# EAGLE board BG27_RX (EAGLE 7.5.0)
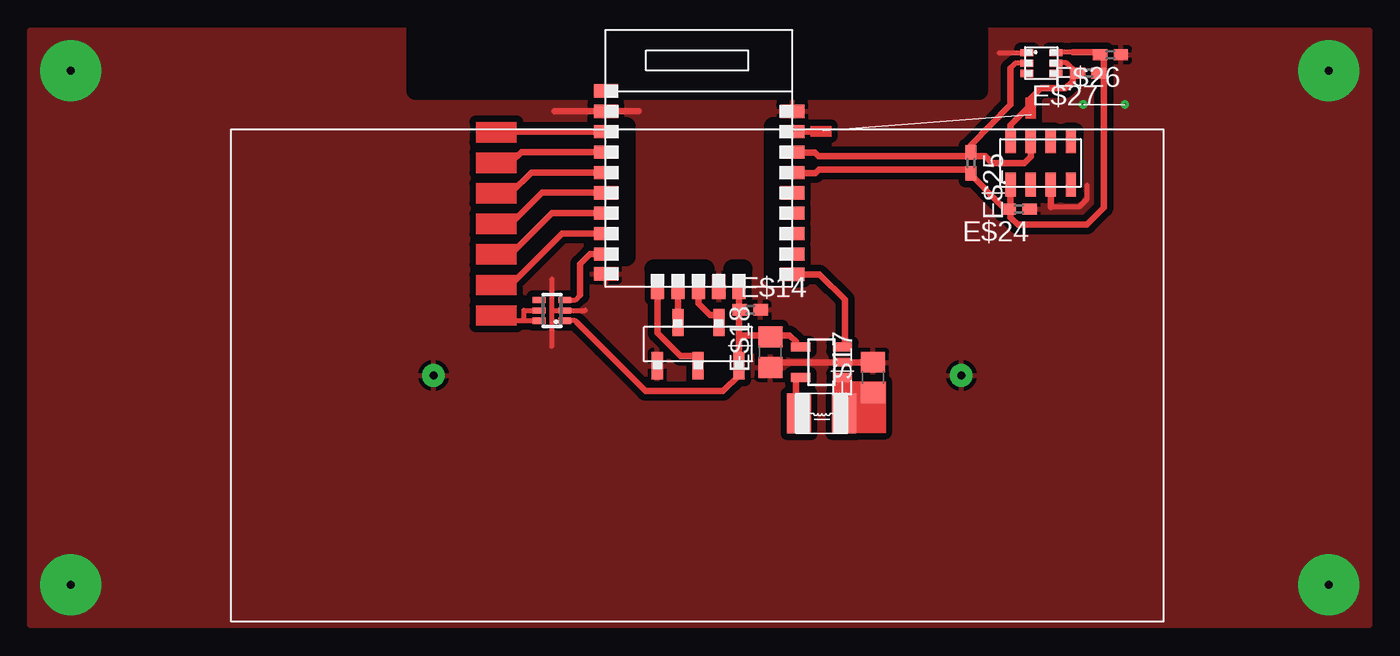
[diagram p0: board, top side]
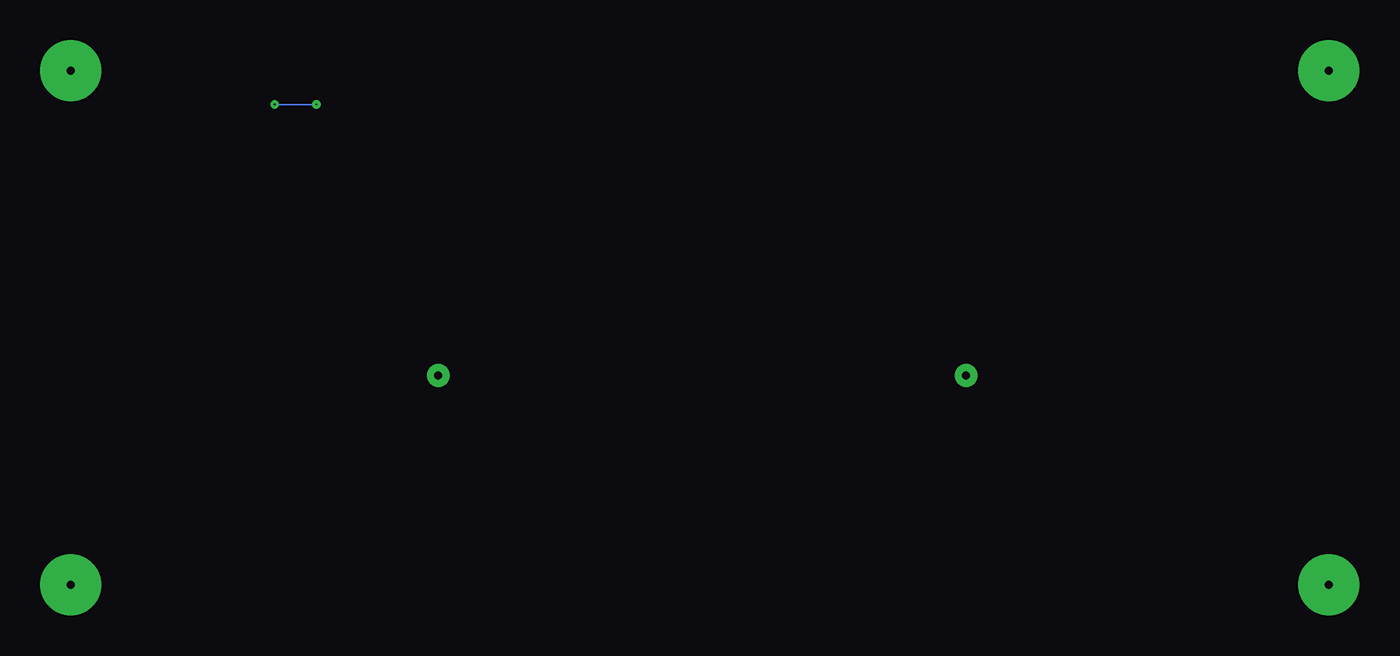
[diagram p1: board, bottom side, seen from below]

No outline drawn. Coordinates in mm, seen from the top.
Copper layers (1*16): Top 0.035mm / dielectric 1.5mm / Bottom 0.035mm
Design rules "default": minimum track width 10mil, minimum drill 24mil, track to track 8mil, track to pad 8mil, pad to pad 8mil, via to via 8mil, smd to smd 8mil, copper to edge 40mil, drill to drill 8mil, minimum pad ring 10mil, minimum via ring 8mil, stop-mask expansion 4mil, vias tented up to drill 0mil, thermal gap 10mil
tRestrict: 9 lines

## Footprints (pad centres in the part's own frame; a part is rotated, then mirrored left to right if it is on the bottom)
HEADER5S = smd 0.7 x 1.7: P$1 0,1.35; P$2 2.55,1.35; P$3 -2.55,1.35; P$4 -1.3,-1.35; P$5 1.25,-1.35
BG22_KIT = smd 1.5 x 0.82: 1 0.02,12.7; 2 0.02,11.43; 3 0.02,10.16; 4 0.02,8.89; 5 0.02,7.62; 6 0.02,6.35; 7 0.02,5.08; 8 0.02,3.81; 9 0.02,2.54; 10 0.02,1.3; 16 11.65,1.27; 17 11.65,2.54; 18 11.65,3.81; 19 11.65,5.08; 20 11.65,6.35; 21 11.65,7.62; 22 11.65,8.89; 23 11.65,10.16; 24 11.65,11.43 | smd 0.82 x 1.5: 11 3.25,0.48; 12 4.52,0.48; 13 5.79,0.48; 14 7.06,0.48; 15 8.33,0.48
C0402 = smd 0.9 x 0.7: 1 -0.65,0; 2 0.65,0
SOT23-5 = smd 0.55 x 1.2: 1 -0.95,-1.3; 2 0,-1.3; 3 0.95,-1.3; 4 0.95,1.3; 5 -0.95,1.3
C0805 = smd 1.3 x 1.5: 1 -0.95,0; 2 0.95,0
LQH32C = smd 1.5 x 2.5: P$1 -1.4,0; P$2 1.4,0
SC70 = smd 0.4 x 0.8: 1 -0.65,-0.8; 2 0,-0.8; 3 0.65,-0.8; 4 0.65,0.8; 5 0,0.8; 6 -0.65,0.8
2XAA = drill 0.5 pad 1.422: P$1 -16.45,0; P$2 16.45,0
VEML6035 = smd 0.8 x 0.45: 1 -0.9,0.65; 2 -0.9,0; 3 -0.9,-0.65; 4 0.9,-0.65; 5 0.9,0; 6 0.9,0.65
MS8607 = smd 1.5 x 0.635: 1 -1.35,1.875; 2 -1.35,0.625; 3 -1.35,-0.625; 4 -1.35,-1.875; 5 1.35,-1.875; 6 1.35,-0.625; 7 1.35,0.625; 8 1.35,1.875

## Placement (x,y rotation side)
E$12  [HEADER5S]  41.65,17.55 180 top
E$13  [BG22_KIT]  35.88,20.64 0 top
E$14  [C0402]  44.9,19.7 0 top
E$16  [SOT23-5]  49.35,16.42 90 top
E$17  [C0805]  52.55,15.47 90 top
E$18  [C0805]  46.15,17.05 90 top
E$19  [LQH32C]  49.35,13.22 180 top
E$20  [SC70]  32.54,19.65 90 top
E$21  [2XAA]  41.6,15.6 0 top
E$22  [VEML6035]  63.04,35.08 0 top
E$24  [C0402]  61.65,25.98 180 top
E$25  [C0402]  58.65,28.85 270 top
E$26  [C0402]  67.35,35.6 180 top
E$27  [C0402]  65.97,34.45 180 top
E$28  [MS8607]  63,28.85 90 top

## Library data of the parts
E$12 E$19 = sb
E$13 = silabs
E$14 E$17 E$18 E$24-E$27 = ref-packages
E$16 = csci381
E$20 = texas
E$21 = battery
E$22 E$28 = sensor

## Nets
GND: E$12.P$2 E$13.10 E$13.14 E$13.24 E$14.2 E$16.2 E$17.2 E$18.1 E$21.P$1 E$21.P$2 E$24.1 E$26.1

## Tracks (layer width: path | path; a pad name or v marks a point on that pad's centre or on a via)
GND  (via drill 0.1 pad 0.25, 0.5 pad 3.81)
  Top 0.305: 32.54,17.43 32.54,21.59 | 32.54,19.65 34.61,19.65 | 60.42,35.73 62.38,35.73 | 63.62,26.1 65.38,26.1 65.9,26.62 65.9,27.45
  Top 0.406: 46.81,16.42 E$17.2 | 32.7,32.07 37.94,32.07 | 63.62,26.1 63.62,27.3
  Bottom 0.1: v65.65,32.5 v68.25,32.5
  other vias: 2.54,2.54 2.54,34.61 80.96,2.54 80.96,34.61
  pour Top (isolate 0.406): 0,37.15 83.5,37.15 83.5,0 0,0
S$17
  Top 0.406: 40.41,18.62 40.41,21.41
S$22
  Top 0.406: 43,19.37 42.38,19.37 41.67,20.07 41.68,20.61
S$23
  Top 0.406: 39.12,20.65 39.12,18.25 40.55,16.82 41.62,16.82
S$24
  Top 0.406: 35.56,24.45 33.18,24.45 30,21.27
S$25
  Top 0.406: 30,23.18 32.54,25.72 35.56,25.72
S$26
  Top 0.406: 30,25.08 31.91,26.99 35.56,26.99
S$27
  Top 0.406: 30,26.99 31.27,28.26 35.56,28.26
S$28
  Top 0.406: 30,28.89 30.64,29.53 35.56,29.53
S$29
  Top 0.406: 30,30.8 35.56,30.8
S$30
  Top 0.406: 47.75,15.32 47.75,13.72
S$31
  Top 0.406: 47.75,17.42 47.75,17.7 47.35,18.11 44.19,18.11
S$32
  Top 0.406: 47.94,21.91 49.21,21.91 50.8,20.32 50.8,17.75
S$33
  Top 0.305: 29.23,19.02 31.43,19.02
S$34
  Top 0.305: 31.43,19.65 30.8,19.65 30.8,19.02
S$35
  Top 0.305: 33.18,20.29 33.97,20.29 34.29,20.61
  Top 0.406: 34.29,20.61 34.29,22.54 34.92,23.18 36.2,23.18
S$36
  Top 0.305: 34.13,18.86 33.97,19.02 33.18,19.02
  Top 0.406: 34.29,18.7 34.13,18.86 35.65,17.35 38.38,14.62 43.21,14.62 44.19,15.6 44.19,20.97
S$37
  Top 0.305: 65,35.75 63.7,35.75
  Top 0.406: 65,35.75 66.95,35.75 66.95,26.07 65.88,25 61.58,25 61.12,25.45 61.12,27.32
S$38
  Top 0.305: 63.7,35.1 64.6,35.1 65,34.7
  Top 0.406: 62.38,32.45 62.38,32.85 63.02,33.5 64.55,33.5 65,33.95 65,34.7
S$39
  Top 0.305: 61.75,35.1 61.45,35.1 61.1,34.75
  Top 0.406: 61.1,32.52 61.1,34.75
S$40
  Top 0.406: 47.7,29.5 48.92,29.5 49.15,29.27 58.65,29.27 58.65,29.95 61.1,32.5
S$41
  Top 0.406: 62.4,29.9 62.4,29.25 62,28.85 59.98,28.85 59.55,29.27 58.75,29.27
S$42
  Top 0.406: 47.85,30.8 49.15,30.8
S$43
  Top 0.406: 48.02,28.23 48.98,28.23 49.17,28.43 58.35,28.43 60.7,26.05
S$44
  Top 0.406: 61.1,30.55 61.1,31.2 62.4,32.5
(copper drawn outside any net)
  shapes: Top area x10

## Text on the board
tDocu: SCL | SDA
